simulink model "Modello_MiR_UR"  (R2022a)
settings: Solver=FixedStepAuto  StartTime=0.0  StopTime=time_s(end,1)  FixedStep=Sim.dt*10  RelTol=1e-3  EnableMultiTasking=on
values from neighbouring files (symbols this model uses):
  a = 0.250    (= 0.25)    [Modello_MiR_UR_script.m]    (also in Modello_MiR_2ruote_script.m; Modello_MiR_6ruote_script.m; Modello_MiR_6ruote_validato_script.m)
  a1 = 0.18265    [Modello_MiR_UR_script.m]    (also in UR_DHtable_e.m = 0; Modello_MiR_2ruote_script.m = deg2rad(5); Modello_MiR_6ruote_script.m = deg2rad(5); Modello_MiR_6ruote_validato_script.m)
  a2 = 0.40857    [Modello_MiR_UR_script.m]    (also in UR_DHtable_e.m = 612; Modello_MiR_2ruote_script.m = deg2rad(25); Modello_MiR_6ruote_script.m = deg2rad(25); Modello_MiR_6ruote_validato_script.m)
  Att_C1 = 0.01    [Modello_MiR_UR_script.m]    (also in Modello_MiR_6ruote_validato_script.m)
  Att_C2 = 0.01    [Modello_MiR_UR_script.m]    (also in Modello_MiR_6ruote_validato_script.m)
  Att_C5 = 0.01    [Modello_MiR_UR_script.m]    (also in Modello_MiR_6ruote_validato_script.m)
  Att_C6 = 0.01    [Modello_MiR_UR_script.m]    (also in Modello_MiR_6ruote_validato_script.m)
  b = 0.1875    [Modello_MiR_UR_script.m]    (also in Modello_MiR_2ruote_script.m; Modello_MiR_6ruote_script.m; Modello_MiR_6ruote_validato_script.m)
  b_caster = 0.07    [Modello_MiR_UR_script.m]    (also in Modello_MiR_2ruote_script.m; Modello_MiR_6ruote_script.m; Modello_MiR_6ruote_validato_script.m)
  bd = 0.205    [Modello_MiR_UR_script.m]    (also in Modello_MiR_2ruote_script.m; Modello_MiR_6ruote_script.m; Modello_MiR_6ruote_validato_script.m)
  F23MIR = @(u) (mv*9.801/4)-(mv*h*u(5)+(mv*9.801/4)*(2*a-b_caster*(cos(u(1))+cos(u(2)))))/(4*a-b_caster*(cos(u(1))+cos(u(2)))+b_caster*(cos(u(3))+cos(u(4))))    [Modello_MiR_UR_script.m]
  F23UR5 = @(u) (u(7)/4)-u(11)    [Modello_MiR_UR_script.m]
  F43MIR = @(u) (1/(2*bd))*(mv*u(6)*h+((mv*h*u(5)+(mv*9.801/4)*(2*a-b_caster*(cos(u(1))+cos(u(2)))))/(4*a-b_caster*(cos(u(1))+cos(u(2)))+b_caster*(cos(u(3))+cos(u(4)))))*(2*bd-b_caster*(sin(u(3))+sin(u(4))))+((mv*9.801/4)-(mv*h*u(5)+(mv*9.801/4)*(2*a-b_caster*(cos(u(1))+cos(u(2)))))/(4*a-b_caster*(cos(u(1))+cos(u(2)))+b_caster*(cos(u(3))+cos(u(4)))))*(2*bd-b_caster*(sin(u(1))+sin(u(2)))))    [Modello_MiR_UR_script.m]
  F43UR5 = @(u) (1/(2*bd))*(u(8) - u(6)*H +u(11)*(2*bd-b_caster*(sin(u(3))+sin(u(4))))+u(12)*(2*bd-b_caster*(sin(u(1))+sin(u(2)))))    [Modello_MiR_UR_script.m]
  F63MIR = @(u) (mv*h*u(5)+(mv*9.801/4)*(2*a-b_caster*(cos(u(1))+cos(u(2)))))/(4*a-b_caster*(cos(u(1))+cos(u(2)))+b_caster*(cos(u(3))+cos(u(4))))    [Modello_MiR_UR_script.m]
  F63UR5 = @(u)(-a*u(7)/2 -u(5)*H -u(9) +(u(7)/4)*(2*a-b_caster*(cos(u(1))+cos(u(2)))))/(4*a-b_caster*(cos(u(1))+cos(u(2)))+b_caster*(cos(u(3))+cos(u(4))))    [Modello_MiR_UR_script.m]
  f_c = 0.29564    [Modello_MiR_UR_script.m]    (also in Modello_MiR_6ruote_validato_script.m)
  f_d3 = 0.35846    [Modello_MiR_UR_script.m]    (also in Modello_MiR_6ruote_validato_script.m)
  f_d4 = 0.2333    [Modello_MiR_UR_script.m]    (also in Modello_MiR_6ruote_validato_script.m)
  fa_c = 0.27474    [Modello_MiR_UR_script.m]    (also in Modello_MiR_6ruote_validato_script.m)
  fa_d3 = 0.3694    [Modello_MiR_UR_script.m]    (also in Modello_MiR_6ruote_validato_script.m)
  fa_d4 = 0.28065    [Modello_MiR_UR_script.m]    (also in Modello_MiR_6ruote_validato_script.m)
  fm_fun = @(u) (u <= -am2 || u >= am2) * 0 + (u > -am2 && u <= -am1) * (- u* Mza/(am2 -am1) - Mza* am2/(am2 -am1)) +           + (u > -am1 && u <= am1) * (Mza * u / am1) + (u > am1 && u < am2) * (Mza * u /(am1 -am2) - Mza * am2 /(am1 - am2))    [Modello_MiR_UR_script.m]    (also in Modello_MiR_6ruote_script.m = @(u) (u <= -am2 | u >= am2)*0 + (u > -am2 && u <= -am1)*(- u; Modello_MiR_6ruote_validato_script.m)
  Hi = 1    [UR5e_data.m]
  Icw_1 = 1/2 * mcw * rc^2    (= 0.002004225735)    [Modello_MiR_UR_script.m]    (also in Modello_MiR_2ruote_script.m; Modello_MiR_6ruote_script.m; Modello_MiR_6ruote_validato_script.m)
  Icw_2 = 1/12 * mcw * ec^2 + 1/4 * mcw * rc^2    (= 0.00104098243873)    [Modello_MiR_UR_script.m]    (also in Modello_MiR_2ruote_script.m; Modello_MiR_6ruote_script.m; Modello_MiR_6ruote_validato_script.m)
  Idw_1 = 1/2 * mdw * rd^2    (= 0.00551836278784)    [Modello_MiR_UR_script.m]    (also in Modello_MiR_2ruote_script.m; Transfer_Function_Gol_Gcl.m = Inertia_vect(jj,1); Modello_MiR_6ruote_script.m; Modello_MiR_6ruote_validato_script.m)
  iMax = 20.7*1.1    (= 22.77)    [Modello_MiR_UR_script.m]    (also in Modello_MiR_2ruote_script.m; Modello_MiR_6ruote_script.m; Modello_MiR_6ruote_validato_script.m)
  Iv = mv * (l^2 + w^2)  / 12    (= 6.75343333333)    [Modello_MiR_UR_script.m]    (also in Modello_MiR_2ruote_script.m; Modello_MiR_6ruote_script.m; Modello_MiR_6ruote_validato_script.m = 8.95033333333)
  Kc = 0.15    [Modello_MiR_UR_script.m]    (also in Modello_MiR_2ruote_script.m; Modello_MiR_6ruote_script.m; Modello_MiR_6ruote_validato_script.m)
  Ki_i = 1    [Modello_MiR_UR_script.m]    (also in Modello_MiR_2ruote_script.m; Modello_MiR_6ruote_script.m; Modello_MiR_6ruote_validato_script.m)
  Ki_v = 1    [Modello_MiR_UR_script.m]    (also in Modello_MiR_2ruote_script.m; Modello_MiR_6ruote_script.m; Modello_MiR_6ruote_validato_script.m)
  kk = 0.00005    (= 5e-05)    [Modello_MiR_UR_script.m]    (also in Modello_MiR_2ruote_script.m; Modello_MiR_6ruote_script.m; Modello_MiR_6ruote_validato_script.m)
  Kp_i = 5    [Modello_MiR_UR_script.m]    (also in Modello_MiR_2ruote_script.m; Modello_MiR_6ruote_script.m; Modello_MiR_6ruote_validato_script.m)
  Kp_v = 5    [Modello_MiR_UR_script.m]    (also in Modello_MiR_2ruote_script.m; Modello_MiR_6ruote_script.m; Modello_MiR_6ruote_validato_script.m)
  kv = 1.5e-6    (= 1.5e-06)    [Modello_MiR_UR_script.m]    (also in Modello_MiR_2ruote_script.m; Modello_MiR_6ruote_script.m; Modello_MiR_6ruote_validato_script.m)
  L = R * tauE    (= 0.00181134822805)    [Modello_MiR_UR_script.m]    (also in Modello_MiR_2ruote_script.m; Modello_MiR_6ruote_script.m; Modello_MiR_6ruote_validato_script.m)
  mcw = rc^2 * pi * ec * rhopoliu + 1    (= 1.02616357632)    [Modello_MiR_UR_script.m]    (also in Modello_MiR_2ruote_script.m; Modello_MiR_6ruote_script.m; Modello_MiR_6ruote_validato_script.m)
  mv = 83    [Modello_MiR_UR_script.m]    (also in Modello_MiR_2ruote_script.m; Modello_MiR_6ruote_script.m; Modello_MiR_6ruote_validato_script.m = 110)
  Phi1_start = psi_mir(1,1)    [Modello_MiR_UR_script.m]    (also in Modello_MiR_6ruote_validato_script.m)
  Phi2_start = psi_mir(1,1)    [Modello_MiR_UR_script.m]    (also in Modello_MiR_6ruote_validato_script.m)
  Phi5_start = psi_mir(1,1)    [Modello_MiR_UR_script.m]    (also in Modello_MiR_6ruote_validato_script.m)
  Phi6_start = psi_mir(1,1)    [Modello_MiR_UR_script.m]    (also in Modello_MiR_6ruote_validato_script.m)
  Psi_start = psi_mir(1,1)    [Modello_MiR_UR_script.m]    (also in Modello_MiR_6ruote_script.m = 1.57079632679; Modello_MiR_6ruote_validato_script.m)
  q0 = [qset.q1.signals.values(1),qset.q2.signals.values(1),qset.q3.signals.values(1),qset.q4.signals.values(1),qset.q5.signals.values(1),qset.q6.signals.values(1)]    [UR5e_simmot.m]
  R = velMax * TorqueMax / (iMax)^2    (= 1.81134822805)    [Modello_MiR_UR_script.m]    (also in Modello_MiR_2ruote_script.m; Modello_MiR_6ruote_script.m; Modello_MiR_6ruote_validato_script.m)
  rap_rid = 10.167    [Modello_MiR_UR_script.m]    (also in Modello_MiR_2ruote_script.m; Modello_MiR_6ruote_script.m; Modello_MiR_6ruote_validato_script.m)
  rc = 0.125/2    (= 0.0625)    [Modello_MiR_UR_script.m]    (also in Modello_MiR_2ruote_script.m; Modello_MiR_6ruote_script.m; Modello_MiR_6ruote_validato_script.m)
  rd = 0.1    [Modello_MiR_UR_script.m]    (also in Modello_MiR_2ruote_script.m; Modello_MiR_6ruote_script.m; Modello_MiR_6ruote_validato_script.m)
  s = 1i*s    [Transfer_Function_Gol_Gcl.m]
  s1 = 0.18987    [Modello_MiR_UR_script.m]    (also in Modello_MiR_2ruote_script.m = 0.2; Modello_MiR_6ruote_script.m = 0.2; Modello_MiR_6ruote_validato_script.m)
  s2 = 0.99533    [Modello_MiR_UR_script.m]    (also in Modello_MiR_2ruote_script.m = 0.8; Modello_MiR_6ruote_script.m = 0.8; Modello_MiR_6ruote_validato_script.m)
  Sx = spline(x ,fl_fun(x),zx)    [Modello_MiR_6ruote_script.m]
  Sy = spline(x ,ft_fun(x),zy)    [Modello_MiR_6ruote_script.m]
  tau_i = 1/(2000*2*pi)    (= 7.95774715459e-05)    [UR5e_data.m]    (also in Transfer_Function_Gol_Gcl.m = Kp_i/Ki_i)
  VaMax = Kc * velMax    (= 41.2443991527)    [Modello_MiR_UR_script.m]    (also in Modello_MiR_2ruote_script.m; Modello_MiR_6ruote_script.m; Modello_MiR_6ruote_validato_script.m)
  X_start = traj(1,1)    [Modello_MiR_UR_script.m]    (also in Modello_MiR_2ruote_script.m = input('Inserire coordinata x iniziale'); Modello_MiR_6ruote_script.m = input('Inserire coordinata x iniziale'); Modello_MiR_6ruote_validato_script.m)
  Y_start = traj(1,2)    [Modello_MiR_UR_script.m]    (also in Modello_MiR_2ruote_script.m = input('Inserire coordinata y iniziale'); Modello_MiR_6ruote_script.m = input('Inserire coordinata y iniziale'); Modello_MiR_6ruote_validato_script.m)
undefined symbols (not defined in the file or in its folder): deg, Driver1, Driver2, Driver3, Driver4, Driver5, Driver6, Ground, J1, J2, J3, J4, J5, J6, kg, L1, L2, L3, L4, L5, L6, m, Motor, N, X, Y, z, Z
libraries: sm_lib x33, nesl_utility x30, slpidlib x10
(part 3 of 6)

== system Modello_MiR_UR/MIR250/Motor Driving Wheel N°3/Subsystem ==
  Thetad_SET : Inport
  Thetad_FB : Inport  Port=2
  iFB : Inport  Port=3
  " 1" : slpidlib/PID Controller  Controller=PID  Form=Parallel  TimeDomain=Continuous-time  UseExternalTs=off  SampleTime=-1  IntegratorMethod=Forward Euler  FilterMethod=Forward Euler  ControllerParametersSource=internal  P=Kp_v  I=Ki_v  UseKiTs=off  D=0  N=1  UseFilter=on  TunerSelectOption=Transfer Function Based (PID Tuner App)  InitialConditionSource=internal  InitialConditionForIntegrator=0  InitialConditionForFilter=0  DifferentiatorICPrevScaledInput=0  ExternalReset=none  TrackingMode=off  Kt=1  LimitOutput=on  SatLimitsSource=internal  UpperSaturationLimit=iMax  LowerSaturationLimit=-iMax  LinearizeAsGain=on  AntiWindupMode=back-calculation  Kb=1  POutMin=[]  POutMax=[]  IOutMin=[]  IOutMax=[]  DOutMin=[]  DOutMax=[]  NOutMin=[]  NOutMax=[]  SumOutMin=[]  SumOutMax=[]  SaturationOutMin=[]  SaturationOutMax=[]  PParamMin=0  PParamMax=[]  IParamMin=0  IParamMax=[]  DParamMin=0  DParamMax=[]  NParamMin=[]  NParamMax=[]  KbParamMin=[]  KbParamMax=[]  KtParamMin=[]  KtParamMax=[]  KbOutMin=[]  KbOutMax=[]  KtOutMin=[]  KtOutMax=[]  IntegratorOutMin=[]  IntegratorOutMax=[]  FilterOutMin=[]  FilterOutMax=[]  SumI1OutMin=[]  SumI1OutMax=[]  SumI2OutMin=[]  SumI2OutMax=[]  SumI3OutMin=[]  SumI3OutMax=[]  SumI4OutMin=[]  SumI4OutMax=[]  SumDOutMin=[]  SumDOutMax=[]  DifferentiatorOutMin=[]  DifferentiatorOutMax=[]  FilterDiffOutCoefMin=[]  FilterDiffOutCoefMax=[]  ReciprocalOutMin=[]  ReciprocalOutMax=[]  SumDenOutMin=[]  SumDenOutMax=[]  SumNumOutMin=[]  SumNumOutMax=[]  DivideOutMin=[]  DivideOutMax=[]  UdiffTsProdOutMin=[]  UdiffTsProdOutMax=[]  NTsProdOutMin=[]  NTsProdOutMax=[]  UintegralTsProdOutMin=[]  UintegralTsProdOutMax=[]  UngainTsProdOutMin=[]  UngainTsProdOutMax=[]  IntegratorContinuousStateAttributes=''  IntegratorStateMustResolveToSignalObject=off  IntegratorRTWStateStorageClass=Auto  FilterContinuousStateAttributes=''  FilterStateMustResolveToSignalObject=off  FilterRTWStateStorageClass=Auto  ParallelPVariant=InternalParameters  IdealPVariant=Disabled  IVariant=InternalParameters  DVariant=InternalParameters  IntegratorVariant=Continuous  SatVariant=Enabled  AWVariant=BackCalculation  PCopyVariant=Disabled  TRVariant=Disabled  FdbkBlocksVariant=Forward  IdealPFdbkVariant=Disabled  SatFdbkVariant=Disabled  DerivativeFilterVariant=ContFilter  NVariant=InternalParameters  NCopyVariant=Disabled  FilterICVariant=InternalICsFilter  IntegratorICVariant=InternalICs  ExternalResetVariant=Disabled  TRSumVariant=Passthrough  SumFdbkVariant=Disabled  SumVariant=Sum_PID  TsampFilterVariant=InternalTs  TsampNgainVariant=Passthrough  TsampIntegralVariant=Passthrough  ExternalSaturationOutDataTypeStr=Inherit: Same as second input  aMode=0
  PID Controller2 : slpidlib/PID Controller  Controller=PID  Form=Parallel  TimeDomain=Continuous-time  UseExternalTs=off  SampleTime=-1  IntegratorMethod=Forward Euler  FilterMethod=Forward Euler  ControllerParametersSource=internal  P=Kp_i  I=Ki_i  UseKiTs=off  D=0  N=100  UseFilter=on  TunerSelectOption=Transfer Function Based (PID Tuner App)  InitialConditionSource=internal  InitialConditionForIntegrator=0  InitialConditionForFilter=0  DifferentiatorICPrevScaledInput=0  ExternalReset=none  TrackingMode=off  Kt=1  LimitOutput=on  SatLimitsSource=internal  UpperSaturationLimit=VaMax  LowerSaturationLimit=-VaMax  LinearizeAsGain=on  AntiWindupMode=back-calculation  Kb=1  POutMin=[]  POutMax=[]  IOutMin=[]  IOutMax=[]  DOutMin=[]  DOutMax=[]  NOutMin=[]  NOutMax=[]  SumOutMin=[]  SumOutMax=[]  SaturationOutMin=[]  SaturationOutMax=[]  PParamMin=[]  PParamMax=[]  IParamMin=[]  IParamMax=[]  DParamMin=[]  DParamMax=[]  NParamMin=[]  NParamMax=[]  KbParamMin=[]  KbParamMax=[]  KtParamMin=[]  KtParamMax=[]  KbOutMin=[]  KbOutMax=[]  KtOutMin=[]  KtOutMax=[]  IntegratorOutMin=[]  IntegratorOutMax=[]  FilterOutMin=[]  FilterOutMax=[]  SumI1OutMin=[]  SumI1OutMax=[]  SumI2OutMin=[]  SumI2OutMax=[]  SumI3OutMin=[]  SumI3OutMax=[]  SumI4OutMin=[]  SumI4OutMax=[]  SumDOutMin=[]  SumDOutMax=[]  DifferentiatorOutMin=[]  DifferentiatorOutMax=[]  FilterDiffOutCoefMin=[]  FilterDiffOutCoefMax=[]  ReciprocalOutMin=[]  ReciprocalOutMax=[]  SumDenOutMin=[]  SumDenOutMax=[]  SumNumOutMin=[]  SumNumOutMax=[]  DivideOutMin=[]  DivideOutMax=[]  UdiffTsProdOutMin=[]  UdiffTsProdOutMax=[]  NTsProdOutMin=[]  NTsProdOutMax=[]  UintegralTsProdOutMin=[]  UintegralTsProdOutMax=[]  UngainTsProdOutMin=[]  UngainTsProdOutMax=[]  IntegratorContinuousStateAttributes=''  IntegratorStateMustResolveToSignalObject=off  IntegratorRTWStateStorageClass=Auto  FilterContinuousStateAttributes=''  FilterStateMustResolveToSignalObject=off  FilterRTWStateStorageClass=Auto  ParallelPVariant=InternalParameters  IdealPVariant=Disabled  IVariant=InternalParameters  DVariant=InternalParameters  IntegratorVariant=Continuous  SatVariant=Enabled  AWVariant=BackCalculation  PCopyVariant=Disabled  TRVariant=Disabled  FdbkBlocksVariant=Forward  IdealPFdbkVariant=Disabled  SatFdbkVariant=Disabled  DerivativeFilterVariant=ContFilter  NVariant=InternalParameters  NCopyVariant=Disabled  FilterICVariant=InternalICsFilter  IntegratorICVariant=InternalICs  ExternalResetVariant=Disabled  TRSumVariant=Passthrough  SumFdbkVariant=Disabled  SumVariant=Sum_PID  TsampFilterVariant=InternalTs  TsampNgainVariant=Passthrough  TsampIntegralVariant=Passthrough  ExternalSaturationOutDataTypeStr=Inherit: Same as second input  aMode=0
  Scope : Scope
  Scope1 : Scope
  Scope2 : Scope
  Scope3 : Scope  NumInputPorts=2
  Sum1 : Sum  Inputs=|+-
  Sum2 : Sum  Inputs=|+-
  VaRif : Outport  VectorParamsAs1DForOutWhenUnconnected=off
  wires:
  Thetad_FB/1 -> Scope3/2, Sum1/2
  " 1"/1 -> Scope2/1, Sum2/1
  PID Controller2/1 -> Scope1/1, VaRif/1
  iFB/1 -> Sum2/2
  Thetad_SET/1 -> Scope3/1, Sum1/1
  Sum1/1 -> " 1"/1, Scope/1
  Sum2/1 -> PID Controller2/1

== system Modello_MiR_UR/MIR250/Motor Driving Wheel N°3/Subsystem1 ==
  VaRif : Inport
  Thetad_FB : Inport  Port=2
  Add : Sum  Inputs=+--
  Gain : Gain  Gain=rap_rid
  Gain1 : Gain  Gain=1/L
  Gain2 : Gain  Gain=Kc
  Gain3 : Gain  Gain=R
  Gain4 : Gain  Gain=Kc
  Integrator : Integrator
  Scope : Scope
  Scope1 : Scope
  Torque Cm : Outport  VectorParamsAs1DForOutWhenUnconnected=off
  iFB : Outport  Port=2  VectorParamsAs1DForOutWhenUnconnected=off
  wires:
  VaRif/1 -> Add/1
  Add/1 -> Gain1/1
  Gain1/1 -> Integrator/1
  Integrator/1 -> Gain4/1, iFB/1, Gain3/1
  Gain3/1 -> Add/3
  Gain4/1 -> Scope1/1, Gain/1
  Thetad_FB/1 -> Gain2/1, Scope/1
  Gain2/1 -> Add/2
  Gain/1 -> Torque Cm/1

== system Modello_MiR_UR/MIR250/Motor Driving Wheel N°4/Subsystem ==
  Thetad_SET : Inport
  Thetad_FB : Inport  Port=2
  iFB : Inport  Port=3
  " " : slpidlib/PID Controller  Controller=PID  Form=Parallel  TimeDomain=Continuous-time  UseExternalTs=off  SampleTime=-1  IntegratorMethod=Forward Euler  FilterMethod=Forward Euler  ControllerParametersSource=internal  P=Kp_v  I=Ki_v  UseKiTs=off  D=0  N=1  UseFilter=on  TunerSelectOption=Transfer Function Based (PID Tuner App)  InitialConditionSource=internal  InitialConditionForIntegrator=0  InitialConditionForFilter=0  DifferentiatorICPrevScaledInput=0  ExternalReset=none  TrackingMode=off  Kt=1  LimitOutput=on  SatLimitsSource=internal  UpperSaturationLimit=iMax  LowerSaturationLimit=-iMax  LinearizeAsGain=on  AntiWindupMode=back-calculation  Kb=1  POutMin=[]  POutMax=[]  IOutMin=[]  IOutMax=[]  DOutMin=[]  DOutMax=[]  NOutMin=[]  NOutMax=[]  SumOutMin=[]  SumOutMax=[]  SaturationOutMin=[]  SaturationOutMax=[]  PParamMin=0  PParamMax=[]  IParamMin=0  IParamMax=[]  DParamMin=0  DParamMax=[]  NParamMin=[]  NParamMax=[]  KbParamMin=[]  KbParamMax=[]  KtParamMin=[]  KtParamMax=[]  KbOutMin=[]  KbOutMax=[]  KtOutMin=[]  KtOutMax=[]  IntegratorOutMin=[]  IntegratorOutMax=[]  FilterOutMin=[]  FilterOutMax=[]  SumI1OutMin=[]  SumI1OutMax=[]  SumI2OutMin=[]  SumI2OutMax=[]  SumI3OutMin=[]  SumI3OutMax=[]  SumI4OutMin=[]  SumI4OutMax=[]  SumDOutMin=[]  SumDOutMax=[]  DifferentiatorOutMin=[]  DifferentiatorOutMax=[]  FilterDiffOutCoefMin=[]  FilterDiffOutCoefMax=[]  ReciprocalOutMin=[]  ReciprocalOutMax=[]  SumDenOutMin=[]  SumDenOutMax=[]  SumNumOutMin=[]  SumNumOutMax=[]  DivideOutMin=[]  DivideOutMax=[]  UdiffTsProdOutMin=[]  UdiffTsProdOutMax=[]  NTsProdOutMin=[]  NTsProdOutMax=[]  UintegralTsProdOutMin=[]  UintegralTsProdOutMax=[]  UngainTsProdOutMin=[]  UngainTsProdOutMax=[]  IntegratorContinuousStateAttributes=''  IntegratorStateMustResolveToSignalObject=off  IntegratorRTWStateStorageClass=Auto  FilterContinuousStateAttributes=''  FilterStateMustResolveToSignalObject=off  FilterRTWStateStorageClass=Auto  ParallelPVariant=InternalParameters  IdealPVariant=Disabled  IVariant=InternalParameters  DVariant=InternalParameters  IntegratorVariant=Continuous  SatVariant=Enabled  AWVariant=BackCalculation  PCopyVariant=Disabled  TRVariant=Disabled  FdbkBlocksVariant=Forward  IdealPFdbkVariant=Disabled  SatFdbkVariant=Disabled  DerivativeFilterVariant=ContFilter  NVariant=InternalParameters  NCopyVariant=Disabled  FilterICVariant=InternalICsFilter  IntegratorICVariant=InternalICs  ExternalResetVariant=Disabled  TRSumVariant=Passthrough  SumFdbkVariant=Disabled  SumVariant=Sum_PID  TsampFilterVariant=InternalTs  TsampNgainVariant=Passthrough  TsampIntegralVariant=Passthrough  ExternalSaturationOutDataTypeStr=Inherit: Same as second input  aMode=0
  PID Controller1 : slpidlib/PID Controller  Controller=PID  Form=Parallel  TimeDomain=Continuous-time  UseExternalTs=off  SampleTime=-1  IntegratorMethod=Forward Euler  FilterMethod=Forward Euler  ControllerParametersSource=internal  P=Kp_i  I=Ki_i  UseKiTs=off  D=0  N=100  UseFilter=on  TunerSelectOption=Transfer Function Based (PID Tuner App)  InitialConditionSource=internal  InitialConditionForIntegrator=0  InitialConditionForFilter=0  DifferentiatorICPrevScaledInput=0  ExternalReset=none  TrackingMode=off  Kt=1  LimitOutput=on  SatLimitsSource=internal  UpperSaturationLimit=VaMax  LowerSaturationLimit=-VaMax  LinearizeAsGain=on  AntiWindupMode=back-calculation  Kb=1  POutMin=[]  POutMax=[]  IOutMin=[]  IOutMax=[]  DOutMin=[]  DOutMax=[]  NOutMin=[]  NOutMax=[]  SumOutMin=[]  SumOutMax=[]  SaturationOutMin=[]  SaturationOutMax=[]  PParamMin=[]  PParamMax=[]  IParamMin=[]  IParamMax=[]  DParamMin=[]  DParamMax=[]  NParamMin=[]  NParamMax=[]  KbParamMin=[]  KbParamMax=[]  KtParamMin=[]  KtParamMax=[]  KbOutMin=[]  KbOutMax=[]  KtOutMin=[]  KtOutMax=[]  IntegratorOutMin=[]  IntegratorOutMax=[]  FilterOutMin=[]  FilterOutMax=[]  SumI1OutMin=[]  SumI1OutMax=[]  SumI2OutMin=[]  SumI2OutMax=[]  SumI3OutMin=[]  SumI3OutMax=[]  SumI4OutMin=[]  SumI4OutMax=[]  SumDOutMin=[]  SumDOutMax=[]  DifferentiatorOutMin=[]  DifferentiatorOutMax=[]  FilterDiffOutCoefMin=[]  FilterDiffOutCoefMax=[]  ReciprocalOutMin=[]  ReciprocalOutMax=[]  SumDenOutMin=[]  SumDenOutMax=[]  SumNumOutMin=[]  SumNumOutMax=[]  DivideOutMin=[]  DivideOutMax=[]  UdiffTsProdOutMin=[]  UdiffTsProdOutMax=[]  NTsProdOutMin=[]  NTsProdOutMax=[]  UintegralTsProdOutMin=[]  UintegralTsProdOutMax=[]  UngainTsProdOutMin=[]  UngainTsProdOutMax=[]  IntegratorContinuousStateAttributes=''  IntegratorStateMustResolveToSignalObject=off  IntegratorRTWStateStorageClass=Auto  FilterContinuousStateAttributes=''  FilterStateMustResolveToSignalObject=off  FilterRTWStateStorageClass=Auto  ParallelPVariant=InternalParameters  IdealPVariant=Disabled  IVariant=InternalParameters  DVariant=InternalParameters  IntegratorVariant=Continuous  SatVariant=Enabled  AWVariant=BackCalculation  PCopyVariant=Disabled  TRVariant=Disabled  FdbkBlocksVariant=Forward  IdealPFdbkVariant=Disabled  SatFdbkVariant=Disabled  DerivativeFilterVariant=ContFilter  NVariant=InternalParameters  NCopyVariant=Disabled  FilterICVariant=InternalICsFilter  IntegratorICVariant=InternalICs  ExternalResetVariant=Disabled  TRSumVariant=Passthrough  SumFdbkVariant=Disabled  SumVariant=Sum_PID  TsampFilterVariant=InternalTs  TsampNgainVariant=Passthrough  TsampIntegralVariant=Passthrough  ExternalSaturationOutDataTypeStr=Inherit: Same as second input  aMode=0
  Scope : Scope  NumInputPorts=2
  Sum1 : Sum  Inputs=|+-
  Sum2 : Sum  Inputs=|+-
  VaRif : Outport  VectorParamsAs1DForOutWhenUnconnected=off
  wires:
  Thetad_FB/1 -> Scope/2, Sum1/2
  " "/1 -> Sum2/1
  PID Controller1/1 -> VaRif/1
  iFB/1 -> Sum2/2
  Thetad_SET/1 -> Scope/1, Sum1/1
  Sum1/1 -> " "/1
  Sum2/1 -> PID Controller1/1

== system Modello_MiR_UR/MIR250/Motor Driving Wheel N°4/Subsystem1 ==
  VaRif : Inport
  Thetad_FB : Inport  Port=2
  Add : Sum  Inputs=+--
  Gain : Gain  Gain=rap_rid
  Gain1 : Gain  Gain=1/L
  Gain2 : Gain  Gain=Kc
  Gain3 : Gain  Gain=R
  Gain4 : Gain  Gain=Kc
  Integrator : Integrator
  Scope : Scope
  Scope1 : Scope
  Torque Cm : Outport  VectorParamsAs1DForOutWhenUnconnected=off
  iFB : Outport  Port=2  VectorParamsAs1DForOutWhenUnconnected=off
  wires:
  VaRif/1 -> Add/1
  Add/1 -> Gain1/1
  Gain1/1 -> Integrator/1
  Integrator/1 -> Gain4/1, Gain3/1, iFB/1
  Gain3/1 -> Add/3
  Thetad_FB/1 -> Gain2/1, Scope/1
  Gain2/1 -> Add/2
  Gain4/1 -> Gain/1
  Gain/1 -> Scope1/1, Torque Cm/1

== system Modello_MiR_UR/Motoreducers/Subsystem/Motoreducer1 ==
  q,qd,qdd : Inport
  Vset : Inport  Port=2
  DC Motor : Subsystem
  Gearbox : Subsystem
  Tu : Outport
  i : Outport  Port=2
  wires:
  Gearbox/2(qm,qdm,qddm) -> DC Motor/2(qm,qdm,qddm)
  DC Motor/1(T) -> Gearbox/1(T)
  Vset/1 -> DC Motor/1(Vset)
  Gearbox/1(Tu) -> Tu/1
  q,qd,qdd/1 -> Gearbox/2(q,qd,qdd)
  DC Motor/2(i) -> i/1

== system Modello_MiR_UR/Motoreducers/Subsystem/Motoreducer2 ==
  q,qd,qdd : Inport
  Vset : Inport  Port=2
  DC Motor : Subsystem
  Gearbox : Subsystem
  Tu : Outport
  i : Outport  Port=2
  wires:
  q,qd,qdd/1 -> Gearbox/2(q,qd,qdd)
  Gearbox/1(Tu) -> Tu/1
  Vset/1 -> DC Motor/1(Vset)
  DC Motor/1(T) -> Gearbox/1(T)
  Gearbox/2(qm,qdm,qddm) -> DC Motor/2(qm,qdm,qddm)
  DC Motor/2(i) -> i/1

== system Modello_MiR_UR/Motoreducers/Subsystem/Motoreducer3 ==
  q,qd,qdd : Inport
  Vset : Inport  Port=2
  DC Motor : Subsystem
  Gearbox : Subsystem
  Tu : Outport
  i : Outport  Port=2
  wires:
  Gearbox/2(qm,qdm,qddm) -> DC Motor/2(qm,qdm,qddm)
  DC Motor/1(T) -> Gearbox/1(T)
  Vset/1 -> DC Motor/1(Vset)
  Gearbox/1(Tu) -> Tu/1
  q,qd,qdd/1 -> Gearbox/2(q,qd,qdd)
  DC Motor/2(i) -> i/1

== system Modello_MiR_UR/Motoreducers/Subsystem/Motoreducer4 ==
  q,qd,qdd : Inport
  Vset : Inport  Port=2
  DC Motor : Subsystem
  Gearbox : Subsystem
  Tu : Outport
  i : Outport  Port=2
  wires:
  q,qd,qdd/1 -> Gearbox/2(q,qd,qdd)
  Gearbox/1(Tu) -> Tu/1
  Vset/1 -> DC Motor/1(Vset)
  DC Motor/1(T) -> Gearbox/1(T)
  Gearbox/2(qm,qdm,qddm) -> DC Motor/2(qm,qdm,qddm)
  DC Motor/2(i) -> i/1

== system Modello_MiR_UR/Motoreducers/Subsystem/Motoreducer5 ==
  q,qd,qdd : Inport
  Vset : Inport  Port=2
  DC Motor : Subsystem
  Gearbox : Subsystem
  Tu : Outport
  i : Outport  Port=2
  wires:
  Gearbox/2(qm,qdm,qddm) -> DC Motor/2(qm,qdm,qddm)
  DC Motor/1(T) -> Gearbox/1(T)
  Vset/1 -> DC Motor/1(Vset)
  Gearbox/1(Tu) -> Tu/1
  q,qd,qdd/1 -> Gearbox/2(q,qd,qdd)
  DC Motor/2(i) -> i/1

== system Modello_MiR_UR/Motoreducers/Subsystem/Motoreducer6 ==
  q,qd,qdd : Inport
  Vset : Inport  Port=2
  DC Motor : Subsystem
  Gearbox : Subsystem
  Tu : Outport
  i : Outport  Port=2
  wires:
  q,qd,qdd/1 -> Gearbox/2(q,qd,qdd)
  Gearbox/1(Tu) -> Tu/1
  Vset/1 -> DC Motor/1(Vset)
  DC Motor/1(T) -> Gearbox/1(T)
  Gearbox/2(qm,qdm,qddm) -> DC Motor/2(qm,qdm,qddm)
  DC Motor/2(i) -> i/1

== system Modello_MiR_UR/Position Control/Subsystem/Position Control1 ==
  qFB,qdFB,qddFB : Inport
  qset,qdset,qddset : Inport  Port=2
  Demux : Demux  Outputs=3
  Demux1 : Demux  Outputs=3
  Gain : Gain  Gain=Driver1.G
  PID Controller : slpidlib/PID Controller  Controller=PI  Form=Parallel  TimeDomain=Continuous-time  UseExternalTs=off  SampleTime=-1  IntegratorMethod=Forward Euler  FilterMethod=Forward Euler  ControllerParametersSource=internal  P=Driver1.P  I=Driver1.I  UseKiTs=off  D=0  N=100  UseFilter=on  TunerSelectOption=Transfer Function Based (PID Tuner App)  InitialConditionSource=internal  InitialConditionForIntegrator=0  InitialConditionForFilter=0  DifferentiatorICPrevScaledInput=0  ExternalReset=none  TrackingMode=off  Kt=1  LimitOutput=off  SatLimitsSource=internal  UpperSaturationLimit=inf  LowerSaturationLimit=-inf  LinearizeAsGain=on  AntiWindupMode=none  Kb=1  POutMin=[]  POutMax=[]  IOutMin=[]  IOutMax=[]  DOutMin=[]  DOutMax=[]  NOutMin=[]  NOutMax=[]  SumOutMin=[]  SumOutMax=[]  SaturationOutMin=[]  SaturationOutMax=[]  PParamMin=[]  PParamMax=[]  IParamMin=[]  IParamMax=[]  DParamMin=[]  DParamMax=[]  NParamMin=[]  NParamMax=[]  KbParamMin=[]  KbParamMax=[]  KtParamMin=[]  KtParamMax=[]  KbOutMin=[]  KbOutMax=[]  KtOutMin=[]  KtOutMax=[]  IntegratorOutMin=[]  IntegratorOutMax=[]  FilterOutMin=[]  FilterOutMax=[]  SumI1OutMin=[]  SumI1OutMax=[]  SumI2OutMin=[]  SumI2OutMax=[]  SumI3OutMin=[]  SumI3OutMax=[]  SumI4OutMin=[]  SumI4OutMax=[]  SumDOutMin=[]  SumDOutMax=[]  DifferentiatorOutMin=[]  DifferentiatorOutMax=[]  FilterDiffOutCoefMin=[]  FilterDiffOutCoefMax=[]  ReciprocalOutMin=[]  ReciprocalOutMax=[]  SumDenOutMin=[]  SumDenOutMax=[]  SumNumOutMin=[]  SumNumOutMax=[]  DivideOutMin=[]  DivideOutMax=[]  UdiffTsProdOutMin=[]  UdiffTsProdOutMax=[]  NTsProdOutMin=[]  NTsProdOutMax=[]  UintegralTsProdOutMin=[]  UintegralTsProdOutMax=[]  UngainTsProdOutMin=[]  UngainTsProdOutMax=[]  IntegratorContinuousStateAttributes=''  IntegratorStateMustResolveToSignalObject=off  IntegratorRTWStateStorageClass=Auto  FilterContinuousStateAttributes=''  FilterStateMustResolveToSignalObject=off  FilterRTWStateStorageClass=Auto  ParallelPVariant=InternalParameters  IdealPVariant=Disabled  IVariant=InternalParameters  DVariant=Disabled  IntegratorVariant=Continuous  SatVariant=Disabled  AWVariant=Passthrough  PCopyVariant=Disabled  TRVariant=Disabled  FdbkBlocksVariant=Forward  IdealPFdbkVariant=Disabled  SatFdbkVariant=Disabled  DerivativeFilterVariant=Disabled  NVariant=Disabled  NCopyVariant=Disabled_SignalSpec  FilterICVariant=Disabled  IntegratorICVariant=InternalICs  ExternalResetVariant=Disabled  TRSumVariant=Passthrough  SumFdbkVariant=Disabled  SumVariant=Sum_PI  TsampFilterVariant=InternalTs  TsampNgainVariant=Passthrough  TsampIntegralVariant=Passthrough  ExternalSaturationOutDataTypeStr=Inherit: Same as second input  aMode=0
  Sum : Sum  Inputs=-+|
  Terminator{,1..3} (4 alike) : Terminator
  Vset : Outport
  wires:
  PID Controller/1 -> Gain/1
  Gain/1 -> Vset/1
  Sum/1 -> PID Controller/1
  Demux1/1 -> Sum/1
  Demux1/3 -> Terminator3/1
  qFB,qdFB,qddFB/1 -> Demux1/1
  Demux1/2 -> Terminator2/1
  Demux/3 -> Terminator1/1
  qset,qdset,qddset/1 -> Demux/1
  Demux/2 -> Terminator/1
  Demux/1 -> Sum/2

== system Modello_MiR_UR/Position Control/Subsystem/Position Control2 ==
  qFB,qdFB,qddFB : Inport
  qset,qdset,qddset : Inport  Port=2
  Demux : Demux  Outputs=3
  Demux1 : Demux  Outputs=3
  Gain : Gain  Gain=Driver2.G
  PID Controller : slpidlib/PID Controller  Controller=PI  Form=Parallel  TimeDomain=Continuous-time  UseExternalTs=off  SampleTime=-1  IntegratorMethod=Forward Euler  FilterMethod=Forward Euler  ControllerParametersSource=internal  P=Driver2.P  I=Driver2.I  UseKiTs=off  D=0  N=100  UseFilter=on  TunerSelectOption=Transfer Function Based (PID Tuner App)  InitialConditionSource=internal  InitialConditionForIntegrator=0  InitialConditionForFilter=0  DifferentiatorICPrevScaledInput=0  ExternalReset=none  TrackingMode=off  Kt=1  LimitOutput=off  SatLimitsSource=internal  UpperSaturationLimit=inf  LowerSaturationLimit=-inf  LinearizeAsGain=on  AntiWindupMode=none  Kb=1  POutMin=[]  POutMax=[]  IOutMin=[]  IOutMax=[]  DOutMin=[]  DOutMax=[]  NOutMin=[]  NOutMax=[]  SumOutMin=[]  SumOutMax=[]  SaturationOutMin=[]  SaturationOutMax=[]  PParamMin=[]  PParamMax=[]  IParamMin=[]  IParamMax=[]  DParamMin=[]  DParamMax=[]  NParamMin=[]  NParamMax=[]  KbParamMin=[]  KbParamMax=[]  KtParamMin=[]  KtParamMax=[]  KbOutMin=[]  KbOutMax=[]  KtOutMin=[]  KtOutMax=[]  IntegratorOutMin=[]  IntegratorOutMax=[]  FilterOutMin=[]  FilterOutMax=[]  SumI1OutMin=[]  SumI1OutMax=[]  SumI2OutMin=[]  SumI2OutMax=[]  SumI3OutMin=[]  SumI3OutMax=[]  SumI4OutMin=[]  SumI4OutMax=[]  SumDOutMin=[]  SumDOutMax=[]  DifferentiatorOutMin=[]  DifferentiatorOutMax=[]  FilterDiffOutCoefMin=[]  FilterDiffOutCoefMax=[]  ReciprocalOutMin=[]  ReciprocalOutMax=[]  SumDenOutMin=[]  SumDenOutMax=[]  SumNumOutMin=[]  SumNumOutMax=[]  DivideOutMin=[]  DivideOutMax=[]  UdiffTsProdOutMin=[]  UdiffTsProdOutMax=[]  NTsProdOutMin=[]  NTsProdOutMax=[]  UintegralTsProdOutMin=[]  UintegralTsProdOutMax=[]  UngainTsProdOutMin=[]  UngainTsProdOutMax=[]  IntegratorContinuousStateAttributes=''  IntegratorStateMustResolveToSignalObject=off  IntegratorRTWStateStorageClass=Auto  FilterContinuousStateAttributes=''  FilterStateMustResolveToSignalObject=off  FilterRTWStateStorageClass=Auto  ParallelPVariant=InternalParameters  IdealPVariant=Disabled  IVariant=InternalParameters  DVariant=Disabled  IntegratorVariant=Continuous  SatVariant=Disabled  AWVariant=Passthrough  PCopyVariant=Disabled  TRVariant=Disabled  FdbkBlocksVariant=Forward  IdealPFdbkVariant=Disabled  SatFdbkVariant=Disabled  DerivativeFilterVariant=Disabled  NVariant=Disabled  NCopyVariant=Disabled_SignalSpec  FilterICVariant=Disabled  IntegratorICVariant=InternalICs  ExternalResetVariant=Disabled  TRSumVariant=Passthrough  SumFdbkVariant=Disabled  SumVariant=Sum_PI  TsampFilterVariant=InternalTs  TsampNgainVariant=Passthrough  TsampIntegralVariant=Passthrough  ExternalSaturationOutDataTypeStr=Inherit: Same as second input  aMode=0
  Sum : Sum  Inputs=-+|
  Terminator{,1..3} (4 alike) : Terminator
  Vset : Outport
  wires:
  Demux/1 -> Sum/2
  Demux/2 -> Terminator/1
  qset,qdset,qddset/1 -> Demux/1
  Demux/3 -> Terminator1/1
  Demux1/2 -> Terminator2/1
  qFB,qdFB,qddFB/1 -> Demux1/1
  Demux1/3 -> Terminator3/1
  Demux1/1 -> Sum/1
  Sum/1 -> PID Controller/1
  Gain/1 -> Vset/1
  PID Controller/1 -> Gain/1

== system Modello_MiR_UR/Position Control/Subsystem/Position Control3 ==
  qFB,qdFB,qddFB : Inport
  qset,qdset,qddset : Inport  Port=2
  Demux : Demux  Outputs=3
  Demux1 : Demux  Outputs=3
  Gain : Gain  Gain=Driver3.G
  PID Controller : slpidlib/PID Controller  Controller=PI  Form=Parallel  TimeDomain=Continuous-time  UseExternalTs=off  SampleTime=-1  IntegratorMethod=Forward Euler  FilterMethod=Forward Euler  ControllerParametersSource=internal  P=Driver3.P  I=Driver3.I  UseKiTs=off  D=0  N=100  UseFilter=on  TunerSelectOption=Transfer Function Based (PID Tuner App)  InitialConditionSource=internal  InitialConditionForIntegrator=0  InitialConditionForFilter=0  DifferentiatorICPrevScaledInput=0  ExternalReset=none  TrackingMode=off  Kt=1  LimitOutput=off  SatLimitsSource=internal  UpperSaturationLimit=inf  LowerSaturationLimit=-inf  LinearizeAsGain=on  AntiWindupMode=none  Kb=1  POutMin=[]  POutMax=[]  IOutMin=[]  IOutMax=[]  DOutMin=[]  DOutMax=[]  NOutMin=[]  NOutMax=[]  SumOutMin=[]  SumOutMax=[]  SaturationOutMin=[]  SaturationOutMax=[]  PParamMin=[]  PParamMax=[]  IParamMin=[]  IParamMax=[]  DParamMin=[]  DParamMax=[]  NParamMin=[]  NParamMax=[]  KbParamMin=[]  KbParamMax=[]  KtParamMin=[]  KtParamMax=[]  KbOutMin=[]  KbOutMax=[]  KtOutMin=[]  KtOutMax=[]  IntegratorOutMin=[]  IntegratorOutMax=[]  FilterOutMin=[]  FilterOutMax=[]  SumI1OutMin=[]  SumI1OutMax=[]  SumI2OutMin=[]  SumI2OutMax=[]  SumI3OutMin=[]  SumI3OutMax=[]  SumI4OutMin=[]  SumI4OutMax=[]  SumDOutMin=[]  SumDOutMax=[]  DifferentiatorOutMin=[]  DifferentiatorOutMax=[]  FilterDiffOutCoefMin=[]  FilterDiffOutCoefMax=[]  ReciprocalOutMin=[]  ReciprocalOutMax=[]  SumDenOutMin=[]  SumDenOutMax=[]  SumNumOutMin=[]  SumNumOutMax=[]  DivideOutMin=[]  DivideOutMax=[]  UdiffTsProdOutMin=[]  UdiffTsProdOutMax=[]  NTsProdOutMin=[]  NTsProdOutMax=[]  UintegralTsProdOutMin=[]  UintegralTsProdOutMax=[]  UngainTsProdOutMin=[]  UngainTsProdOutMax=[]  IntegratorContinuousStateAttributes=''  IntegratorStateMustResolveToSignalObject=off  IntegratorRTWStateStorageClass=Auto  FilterContinuousStateAttributes=''  FilterStateMustResolveToSignalObject=off  FilterRTWStateStorageClass=Auto  ParallelPVariant=InternalParameters  IdealPVariant=Disabled  IVariant=InternalParameters  DVariant=Disabled  IntegratorVariant=Continuous  SatVariant=Disabled  AWVariant=Passthrough  PCopyVariant=Disabled  TRVariant=Disabled  FdbkBlocksVariant=Forward  IdealPFdbkVariant=Disabled  SatFdbkVariant=Disabled  DerivativeFilterVariant=Disabled  NVariant=Disabled  NCopyVariant=Disabled_SignalSpec  FilterICVariant=Disabled  IntegratorICVariant=InternalICs  ExternalResetVariant=Disabled  TRSumVariant=Passthrough  SumFdbkVariant=Disabled  SumVariant=Sum_PI  TsampFilterVariant=InternalTs  TsampNgainVariant=Passthrough  TsampIntegralVariant=Passthrough  ExternalSaturationOutDataTypeStr=Inherit: Same as second input  aMode=0
  Sum : Sum  Inputs=-+|
  Terminator{,1..3} (4 alike) : Terminator
  Vset : Outport
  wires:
  PID Controller/1 -> Gain/1
  Gain/1 -> Vset/1
  Sum/1 -> PID Controller/1
  Demux1/1 -> Sum/1
  Demux1/3 -> Terminator3/1
  qFB,qdFB,qddFB/1 -> Demux1/1
  Demux1/2 -> Terminator2/1
  Demux/3 -> Terminator1/1
  qset,qdset,qddset/1 -> Demux/1
  Demux/2 -> Terminator/1
  Demux/1 -> Sum/2

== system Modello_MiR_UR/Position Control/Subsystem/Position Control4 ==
  qFB,qdFB,qddFB : Inport
  qset,qdset,qddset : Inport  Port=2
  Demux : Demux  Outputs=3
  Demux1 : Demux  Outputs=3
  Gain : Gain  Gain=Driver4.G
  PID Controller : slpidlib/PID Controller  Controller=PI  Form=Parallel  TimeDomain=Continuous-time  UseExternalTs=off  SampleTime=-1  IntegratorMethod=Forward Euler  FilterMethod=Forward Euler  ControllerParametersSource=internal  P=Driver4.P  I=Driver4.I  UseKiTs=off  D=0  N=100  UseFilter=on  TunerSelectOption=Transfer Function Based (PID Tuner App)  InitialConditionSource=internal  InitialConditionForIntegrator=0  InitialConditionForFilter=0  DifferentiatorICPrevScaledInput=0  ExternalReset=none  TrackingMode=off  Kt=1  LimitOutput=off  SatLimitsSource=internal  UpperSaturationLimit=inf  LowerSaturationLimit=-inf  LinearizeAsGain=on  AntiWindupMode=none  Kb=1  POutMin=[]  POutMax=[]  IOutMin=[]  IOutMax=[]  DOutMin=[]  DOutMax=[]  NOutMin=[]  NOutMax=[]  SumOutMin=[]  SumOutMax=[]  SaturationOutMin=[]  SaturationOutMax=[]  PParamMin=[]  PParamMax=[]  IParamMin=[]  IParamMax=[]  DParamMin=[]  DParamMax=[]  NParamMin=[]  NParamMax=[]  KbParamMin=[]  KbParamMax=[]  KtParamMin=[]  KtParamMax=[]  KbOutMin=[]  KbOutMax=[]  KtOutMin=[]  KtOutMax=[]  IntegratorOutMin=[]  IntegratorOutMax=[]  FilterOutMin=[]  FilterOutMax=[]  SumI1OutMin=[]  SumI1OutMax=[]  SumI2OutMin=[]  SumI2OutMax=[]  SumI3OutMin=[]  SumI3OutMax=[]  SumI4OutMin=[]  SumI4OutMax=[]  SumDOutMin=[]  SumDOutMax=[]  DifferentiatorOutMin=[]  DifferentiatorOutMax=[]  FilterDiffOutCoefMin=[]  FilterDiffOutCoefMax=[]  ReciprocalOutMin=[]  ReciprocalOutMax=[]  SumDenOutMin=[]  SumDenOutMax=[]  SumNumOutMin=[]  SumNumOutMax=[]  DivideOutMin=[]  DivideOutMax=[]  UdiffTsProdOutMin=[]  UdiffTsProdOutMax=[]  NTsProdOutMin=[]  NTsProdOutMax=[]  UintegralTsProdOutMin=[]  UintegralTsProdOutMax=[]  UngainTsProdOutMin=[]  UngainTsProdOutMax=[]  IntegratorContinuousStateAttributes=''  IntegratorStateMustResolveToSignalObject=off  IntegratorRTWStateStorageClass=Auto  FilterContinuousStateAttributes=''  FilterStateMustResolveToSignalObject=off  FilterRTWStateStorageClass=Auto  ParallelPVariant=InternalParameters  IdealPVariant=Disabled  IVariant=InternalParameters  DVariant=Disabled  IntegratorVariant=Continuous  SatVariant=Disabled  AWVariant=Passthrough  PCopyVariant=Disabled  TRVariant=Disabled  FdbkBlocksVariant=Forward  IdealPFdbkVariant=Disabled  SatFdbkVariant=Disabled  DerivativeFilterVariant=Disabled  NVariant=Disabled  NCopyVariant=Disabled_SignalSpec  FilterICVariant=Disabled  IntegratorICVariant=InternalICs  ExternalResetVariant=Disabled  TRSumVariant=Passthrough  SumFdbkVariant=Disabled  SumVariant=Sum_PI  TsampFilterVariant=InternalTs  TsampNgainVariant=Passthrough  TsampIntegralVariant=Passthrough  ExternalSaturationOutDataTypeStr=Inherit: Same as second input  aMode=0
  Sum : Sum  Inputs=-+|
  Terminator{,1..3} (4 alike) : Terminator
  Vset : Outport
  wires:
  Demux/1 -> Sum/2
  Demux/2 -> Terminator/1
  qset,qdset,qddset/1 -> Demux/1
  Demux/3 -> Terminator1/1
  Demux1/2 -> Terminator2/1
  qFB,qdFB,qddFB/1 -> Demux1/1
  Demux1/3 -> Terminator3/1
  Demux1/1 -> Sum/1
  Sum/1 -> PID Controller/1
  Gain/1 -> Vset/1
  PID Controller/1 -> Gain/1

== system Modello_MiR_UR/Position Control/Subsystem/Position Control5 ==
  qFB,qdFB,qddFB : Inport
  qset,qdset,qddset : Inport  Port=2
  Demux : Demux  Outputs=3
  Demux1 : Demux  Outputs=3
  Gain : Gain  Gain=Driver5.G
  PID Controller : slpidlib/PID Controller  Controller=PI  Form=Parallel  TimeDomain=Continuous-time  UseExternalTs=off  SampleTime=-1  IntegratorMethod=Forward Euler  FilterMethod=Forward Euler  ControllerParametersSource=internal  P=Driver5.P  I=Driver5.I  UseKiTs=off  D=0  N=100  UseFilter=on  TunerSelectOption=Transfer Function Based (PID Tuner App)  InitialConditionSource=internal  InitialConditionForIntegrator=0  InitialConditionForFilter=0  DifferentiatorICPrevScaledInput=0  ExternalReset=none  TrackingMode=off  Kt=1  LimitOutput=off  SatLimitsSource=internal  UpperSaturationLimit=inf  LowerSaturationLimit=-inf  LinearizeAsGain=on  AntiWindupMode=none  Kb=1  POutMin=[]  POutMax=[]  IOutMin=[]  IOutMax=[]  DOutMin=[]  DOutMax=[]  NOutMin=[]  NOutMax=[]  SumOutMin=[]  SumOutMax=[]  SaturationOutMin=[]  SaturationOutMax=[]  PParamMin=[]  PParamMax=[]  IParamMin=[]  IParamMax=[]  DParamMin=[]  DParamMax=[]  NParamMin=[]  NParamMax=[]  KbParamMin=[]  KbParamMax=[]  KtParamMin=[]  KtParamMax=[]  KbOutMin=[]  KbOutMax=[]  KtOutMin=[]  KtOutMax=[]  IntegratorOutMin=[]  IntegratorOutMax=[]  FilterOutMin=[]  FilterOutMax=[]  SumI1OutMin=[]  SumI1OutMax=[]  SumI2OutMin=[]  SumI2OutMax=[]  SumI3OutMin=[]  SumI3OutMax=[]  SumI4OutMin=[]  SumI4OutMax=[]  SumDOutMin=[]  SumDOutMax=[]  DifferentiatorOutMin=[]  DifferentiatorOutMax=[]  FilterDiffOutCoefMin=[]  FilterDiffOutCoefMax=[]  ReciprocalOutMin=[]  ReciprocalOutMax=[]  SumDenOutMin=[]  SumDenOutMax=[]  SumNumOutMin=[]  SumNumOutMax=[]  DivideOutMin=[]  DivideOutMax=[]  UdiffTsProdOutMin=[]  UdiffTsProdOutMax=[]  NTsProdOutMin=[]  NTsProdOutMax=[]  UintegralTsProdOutMin=[]  UintegralTsProdOutMax=[]  UngainTsProdOutMin=[]  UngainTsProdOutMax=[]  IntegratorContinuousStateAttributes=''  IntegratorStateMustResolveToSignalObject=off  IntegratorRTWStateStorageClass=Auto  FilterContinuousStateAttributes=''  FilterStateMustResolveToSignalObject=off  FilterRTWStateStorageClass=Auto  ParallelPVariant=InternalParameters  IdealPVariant=Disabled  IVariant=InternalParameters  DVariant=Disabled  IntegratorVariant=Continuous  SatVariant=Disabled  AWVariant=Passthrough  PCopyVariant=Disabled  TRVariant=Disabled  FdbkBlocksVariant=Forward  IdealPFdbkVariant=Disabled  SatFdbkVariant=Disabled  DerivativeFilterVariant=Disabled  NVariant=Disabled  NCopyVariant=Disabled_SignalSpec  FilterICVariant=Disabled  IntegratorICVariant=InternalICs  ExternalResetVariant=Disabled  TRSumVariant=Passthrough  SumFdbkVariant=Disabled  SumVariant=Sum_PI  TsampFilterVariant=InternalTs  TsampNgainVariant=Passthrough  TsampIntegralVariant=Passthrough  ExternalSaturationOutDataTypeStr=Inherit: Same as second input  aMode=0
  Sum : Sum  Inputs=-+|
  Terminator{,1..3} (4 alike) : Terminator
  Vset : Outport
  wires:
  PID Controller/1 -> Gain/1
  Gain/1 -> Vset/1
  Sum/1 -> PID Controller/1
  Demux1/1 -> Sum/1
  Demux1/3 -> Terminator3/1
  qFB,qdFB,qddFB/1 -> Demux1/1
  Demux1/2 -> Terminator2/1
  Demux/3 -> Terminator1/1
  qset,qdset,qddset/1 -> Demux/1
  Demux/2 -> Terminator/1
  Demux/1 -> Sum/2

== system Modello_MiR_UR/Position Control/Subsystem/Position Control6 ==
  qFB,qdFB,qddFB : Inport
  qset,qdset,qddset : Inport  Port=2
  Demux : Demux  Outputs=3
  Demux1 : Demux  Outputs=3
  Gain : Gain  Gain=Driver6.G
  PID Controller : slpidlib/PID Controller  Controller=PI  Form=Parallel  TimeDomain=Continuous-time  UseExternalTs=off  SampleTime=-1  IntegratorMethod=Forward Euler  FilterMethod=Forward Euler  ControllerParametersSource=internal  P=Driver6.P  I=Driver6.I  UseKiTs=off  D=0  N=100  UseFilter=on  TunerSelectOption=Transfer Function Based (PID Tuner App)  InitialConditionSource=internal  InitialConditionForIntegrator=0  InitialConditionForFilter=0  DifferentiatorICPrevScaledInput=0  ExternalReset=none  TrackingMode=off  Kt=1  LimitOutput=off  SatLimitsSource=internal  UpperSaturationLimit=inf  LowerSaturationLimit=-inf  LinearizeAsGain=on  AntiWindupMode=none  Kb=1  POutMin=[]  POutMax=[]  IOutMin=[]  IOutMax=[]  DOutMin=[]  DOutMax=[]  NOutMin=[]  NOutMax=[]  SumOutMin=[]  SumOutMax=[]  SaturationOutMin=[]  SaturationOutMax=[]  PParamMin=[]  PParamMax=[]  IParamMin=[]  IParamMax=[]  DParamMin=[]  DParamMax=[]  NParamMin=[]  NParamMax=[]  KbParamMin=[]  KbParamMax=[]  KtParamMin=[]  KtParamMax=[]  KbOutMin=[]  KbOutMax=[]  KtOutMin=[]  KtOutMax=[]  IntegratorOutMin=[]  IntegratorOutMax=[]  FilterOutMin=[]  FilterOutMax=[]  SumI1OutMin=[]  SumI1OutMax=[]  SumI2OutMin=[]  SumI2OutMax=[]  SumI3OutMin=[]  SumI3OutMax=[]  SumI4OutMin=[]  SumI4OutMax=[]  SumDOutMin=[]  SumDOutMax=[]  DifferentiatorOutMin=[]  DifferentiatorOutMax=[]  FilterDiffOutCoefMin=[]  FilterDiffOutCoefMax=[]  ReciprocalOutMin=[]  ReciprocalOutMax=[]  SumDenOutMin=[]  SumDenOutMax=[]  SumNumOutMin=[]  SumNumOutMax=[]  DivideOutMin=[]  DivideOutMax=[]  UdiffTsProdOutMin=[]  UdiffTsProdOutMax=[]  NTsProdOutMin=[]  NTsProdOutMax=[]  UintegralTsProdOutMin=[]  UintegralTsProdOutMax=[]  UngainTsProdOutMin=[]  UngainTsProdOutMax=[]  IntegratorContinuousStateAttributes=''  IntegratorStateMustResolveToSignalObject=off  IntegratorRTWStateStorageClass=Auto  FilterContinuousStateAttributes=''  FilterStateMustResolveToSignalObject=off  FilterRTWStateStorageClass=Auto  ParallelPVariant=InternalParameters  IdealPVariant=Disabled  IVariant=InternalParameters  DVariant=Disabled  IntegratorVariant=Continuous  SatVariant=Disabled  AWVariant=Passthrough  PCopyVariant=Disabled  TRVariant=Disabled  FdbkBlocksVariant=Forward  IdealPFdbkVariant=Disabled  SatFdbkVariant=Disabled  DerivativeFilterVariant=Disabled  NVariant=Disabled  NCopyVariant=Disabled_SignalSpec  FilterICVariant=Disabled  IntegratorICVariant=InternalICs  ExternalResetVariant=Disabled  TRSumVariant=Passthrough  SumFdbkVariant=Disabled  SumVariant=Sum_PI  TsampFilterVariant=InternalTs  TsampNgainVariant=Passthrough  TsampIntegralVariant=Passthrough  ExternalSaturationOutDataTypeStr=Inherit: Same as second input  aMode=0
  Sum : Sum  Inputs=-+|
  Terminator{,1..3} (4 alike) : Terminator
  Vset : Outport
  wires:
  Demux/1 -> Sum/2
  Demux/2 -> Terminator/1
  qset,qdset,qddset/1 -> Demux/1
  Demux/3 -> Terminator1/1
  Demux1/2 -> Terminator2/1
  qFB,qdFB,qddFB/1 -> Demux1/1
  Demux1/3 -> Terminator3/1
  Demux1/1 -> Sum/1
  Sum/1 -> PID Controller/1
  Gain/1 -> Vset/1
  PID Controller/1 -> Gain/1

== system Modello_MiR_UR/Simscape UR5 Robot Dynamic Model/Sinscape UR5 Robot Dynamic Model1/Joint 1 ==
  T1 : Inport
  A_01*E_01 : sm_lib/Frames and Transforms/Rigid Transform  TranslationMethod=None  TranslationStandardOffset=0  TranslationLengthUnit=mm  TranslationStandardAxis=+Z  TranslationCartesianOffset=A01t  TranslationROffset=0  TranslationROffsetUnits=m  TranslationZOffset=0  TranslationZOffsetUnits=m  TranslationThetaOffset=0  TranslationThetaOffsetUnits=deg  RotationMethod=RotationMatrix  RotationAngleUnits=deg  RotationStandardAxis=+Z  RotationAngle=0.0  RotationArbitraryAxis=[0 0 1]  FollAlignAxisA=+X  BaseAlignAxisA=+Y  FollAlignAxisB=+Y  BaseAlignAxisB=+Z  RotationSequenceAxes=FollowerAxes  RotationSequence=XYX  RotationSequenceAngles=[0 0 0]  RotationSequenceAnglesUnits=deg  RotationMatrix=A01r
  A_01*E_1 : sm_lib/Frames and Transforms/Rigid Transform  TranslationMethod=Cartesian  TranslationStandardOffset=0  TranslationLengthUnit=mm  TranslationStandardAxis=+Z  TranslationCartesianOffset=A01t  TranslationROffset=0  TranslationROffsetUnits=m  TranslationZOffset=0  TranslationZOffsetUnits=m  TranslationThetaOffset=0  TranslationThetaOffsetUnits=deg  RotationMethod=None  RotationAngleUnits=deg  RotationStandardAxis=+Z  RotationAngle=0.0  RotationArbitraryAxis=[0 0 1]  FollAlignAxisA=+X  BaseAlignAxisA=+Y  FollAlignAxisB=+Y  BaseAlignAxisB=+Z  RotationSequenceAxes=FollowerAxes  RotationSequence=XYX  RotationSequenceAngles=[0 0 0]  RotationSequenceAnglesUnits=deg  RotationMatrix=A01r
  Mux : Mux  Inputs=3
  PS-Simulink Converter1 : nesl_utility/PS-Simulink Converter  PhysicalDomain=network_engine_domain  SubClassName=ps_output  LeftPortType=input  RightPortType=output  PseudoPeriodic=off  Frequencies=[]  VectorFormat=1-D array  Unit=1  AffineConversion=off
  PS-Simulink Converter2 : nesl_utility/PS-Simulink Converter  PhysicalDomain=network_engine_domain  SubClassName=ps_output  LeftPortType=input  RightPortType=output  PseudoPeriodic=off  Frequencies=[]  VectorFormat=1-D array  Unit=1  AffineConversion=off
  PS-Simulink Converter7 : nesl_utility/PS-Simulink Converter  PhysicalDomain=network_engine_domain  SubClassName=ps_output  LeftPortType=input  RightPortType=output  PseudoPeriodic=off  Frequencies=[]  VectorFormat=1-D array  Unit=1  AffineConversion=off
  Revolute Joint1 : sm_lib/Joints/Revolute Joint  JointMode=Normal  SenseConstraintForce=off  SenseConstraintForceX=off  SenseConstraintForceY=off  SenseConstraintForceZ=off  SenseConstraintTorque=off  SenseConstraintTorqueX=off  SenseConstraintTorqueY=off  SenseConstraintTorqueZ=off  SenseTotalForce=off  SenseTotalForceX=off  SenseTotalForceY=off  SenseTotalForceZ=off  SenseTotalTorque=off  SenseTotalTorqueX=off  SenseTotalTorqueY=off  SenseTotalTorqueZ=off  CompositeWrenchDir=FollowerOnBase  CompositeWrenchFrame=BaseFrame  EquilibriumPosition=0  EquilibriumPositionUnits=deg  SpringStiffness=0  SpringStiffnessUnits=N*m/deg  DampingCoefficient=0  DampingCoefficientUnits=N*m/(deg/s)  TorqueActuationMode=InputTorque  MotionActuationMode=ComputedMotion  SensePosition=on  SenseVelocity=on  SenseAcceleration=on  SenseTorqueForce=off  SenseLowerLimitTorqueForce=off  SenseUpperLimitTorqueForce=off  LowerLimitSpecify=on  LowerLimitBound=-J1.al  LowerLimitBoundUnits=deg  LowerLimitStiffness=1e4  LowerLimitStiffnessUnits=N*m/deg  LowerLimitDamping=10  LowerLimitDampingUnits=N*m/(deg/s)  LowerLimitTransitionRegionWidth=0.1  LowerLimitTransitionRegionWidthUnits=deg  UpperLimitSpecify=on  UpperLimitBound=J1.al  UpperLimitBoundUnits=deg  UpperLimitStiffness=1e4  UpperLimitStiffnessUnits=N*m/deg  UpperLimitDamping=10  UpperLimitDampingUnits=N*m/(deg/s)  UpperLimitTransitionRegionWidth=0.1  UpperLimitTransitionRegionWidthUnits=deg  PositionTargetSpecify=on  PositionTargetPriority=High  PositionTargetValue=q0(1)  PositionTargetValueUnits=rad  VelocityTargetSpecify=off  VelocityTargetPriority=High  VelocityTargetValue=0  VelocityTargetValueUnits=deg/s
  Simulink-PS Converter : nesl_utility/Simulink-PS Converter  PhysicalDomain=network_engine_domain  SubClassName=ps_input  LeftPortType=input  RightPortType=output  PseudoPeriodic=off  Frequencies=[]  NoiseDistribution=none  NoiseParameters=[]  Unit=1  AffineConversion=off  FilteringAndDerivatives=provide  SimscapeFilterOrder=1  InputFilterTimeConstant=0.001  UdotUserProvided=0
  Link 0 : PMIOPort  Side=Left
  Link 1 : PMIOPort  Port=2  Side=Right
  q1,qd1,qdd1 : Outport
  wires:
  T1/1 -> Simulink-PS Converter/1
  PS-Simulink Converter7/1 -> Mux/2
  Mux/1 -> q1,qd1,qdd1/1
  PS-Simulink Converter1/1 -> Mux/1
  PS-Simulink Converter2/1 -> Mux/3
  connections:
  Revolute Joint1/LConn1 -- A_01*E_1/RConn1
  A_01*E_1/LConn1 -- A_01*E_01/RConn1
  Revolute Joint1/RConn1 -- Link 1/RConn1
  Link 0/RConn1 -- A_01*E_01/LConn1
  Simulink-PS Converter/RConn1 -- Revolute Joint1/LConn2
  Revolute Joint1/RConn2 -- PS-Simulink Converter1/LConn1
  Revolute Joint1/RConn3 -- PS-Simulink Converter7/LConn1
  Revolute Joint1/RConn4 -- PS-Simulink Converter2/LConn1
